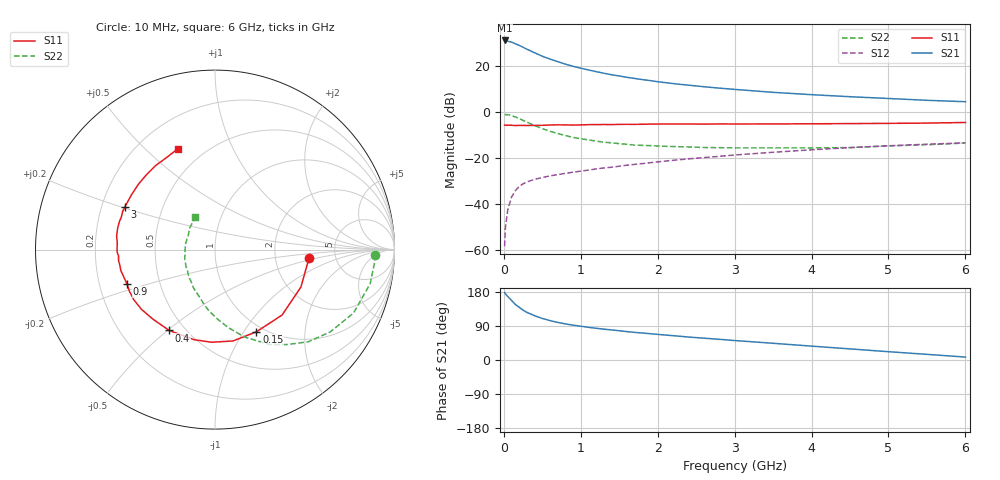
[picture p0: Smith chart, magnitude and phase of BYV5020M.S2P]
! SIEMENS Small Signal Semiconductors
! BFY420
! Si NPN RF SIEGET Grounded Emitter Transistor in MICRO-X
! VCE = 0.5 V  IC = 20 mA
! Common Emitter S-Parameters:  October  1996
# GHz  S  MA  R  50
!  f  S11  S21  S12  S22
! GHz  MAG  ANG  MAG  ANG  MAG  ANG  MAG  ANG
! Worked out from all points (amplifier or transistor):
!   36 points, 10 MHz to 6 GHz, reference 50 ohm
!   highest |S21| = 31.3 dB at 10 MHz (marker M1)
!   |S21| within 3 dB of that: start of sweep to 251.4 MHz
!   unconditionally stable (mu >= 1): start of sweep to 14.82 MHz; 1.501 GHz to end of sweep
!   at 250 MHz: K = 0.34, MSG = 29.8 dB, |S12| = -31.2 dB
!   at 1.4 GHz: K = 0.99, MSG = 20.2 dB, |S12| = -24.0 dB
!   at 6 GHz: K = 1.13, MAG = 6.8 dB, |S12| = -13.3 dB
!   S11 on the Smith chart (normalised r, x): 10 MHz: 3.15, -0.42; 150 MHz: 0.92, -1.14; 400 MHz: 0.41, -0.51; 900 MHz: 0.32, -0.17; 3 GHz: 0.30, +0.21; 6 GHz: 0.36, +0.63
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0.01  0.5253 -5.3  36.87 178.3  0.0012 92.2  0.8915 -1.9
0.02  0.52 -9.8  36.47 174.6  0.003 84.5  0.8922 -4.5
0.05  0.5222 -23.5  35.45 167.7  0.0073 81.6  0.8854 -12.3
0.1  0.5221 -44.3  33.96 157.3  0.0141 75.2  0.8489 -24.6
0.15  0.5128 -63.2  31.19 146.5  0.0195 66.1  0.7891 -35.5
0.2  0.5189 -78.9  28.82 139.1  0.0241 61.0  0.7311 -44.6
0.25  0.5164 -92.2  26.18 131.4  0.0275 56.9  0.6632 -52.9
0.3  0.5153 -103.0  23.76 125.7  0.0303 54.7  0.6111 -60.0
0.4  0.5176 -119.5  19.86 116.9  0.0345 50.6  0.5136 -71.4
0.5  0.5193 -131.7  16.7 109.6  0.0377 48.3  0.4399 -80.5
0.6  0.5279 -140.8  14.47 104.0  0.041 47.2  0.3852 -88.3
0.7  0.5317 -148.4  12.72 99.2  0.0436 47.8  0.3441 -95.4
0.9  0.5262 -158.6  10.07 92.0  0.0493 47.5  0.2829 -106.7
1.1  0.5373 -167.3  8.383 86.2  0.0548 48.2  0.25 -117.5
1.3  0.5409 -173.4  7.106 81.4  0.061 48.4  0.2225 -126.6
1.6  0.5459 179.0  5.786 74.9  0.0701 48.7  0.2002 -139.3
2.2  0.5554 167.3  4.228 64.2  0.0895 47.5  0.1789 -158.1
3  0.5554 154.6  3.158 51.4  0.1169 43.2  0.1673 -177.9
3.5  0.5565 146.9  2.724 44.1  0.1341 39.8  0.1675 171.4
4.5  0.5658 132.4  2.185 29.3  0.1693 30.5  0.1699 150.4
5.5  0.5809 117.0  1.824 14.9  0.2012 20.0  0.1959 129.7
6  0.5989 110.2  1.701 7.7  0.2152 14.7  0.2135 121.6
